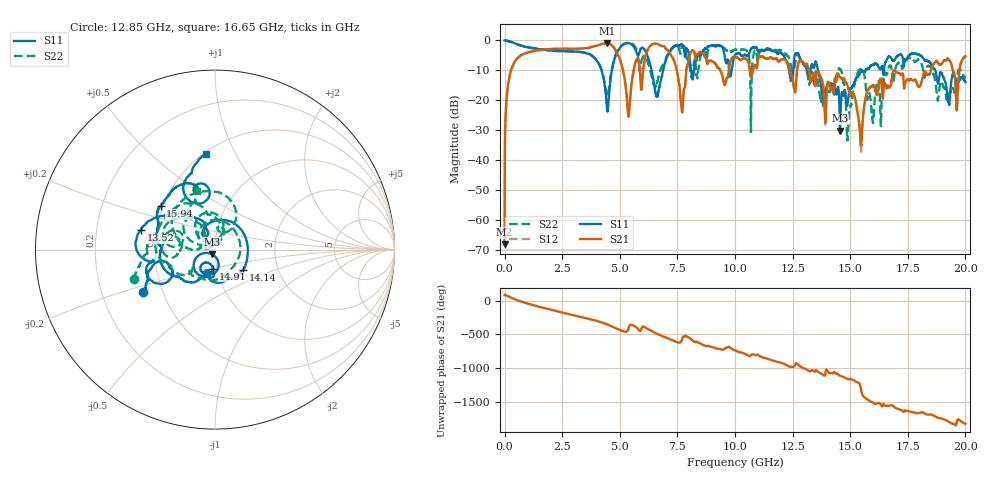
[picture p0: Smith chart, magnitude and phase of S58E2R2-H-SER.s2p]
!{S58E2R2}
!Johanson Technology Inc.
!www.johansontechnology.com
!Test Board Conditions:
!Substrate Type  RO4350B
!Substrate Thickness  60 mil
!Substrate Dk  3.66
!TL Type: GCPW
!TL Trace Width  115 mil
!TL Gap  52 mil
!Electrode orientation  Horizontal
!DUT TOPOLOGY	SERIES
!Mounting Pad LxW  55x428 mil
! Created Tue Apr 13 22:29:26 2021
# hz S ma R 50
! 2 Port Network Data from SP1.SP block
! freq  magS11  angS11  magS21  angS21  magS12  angS12  magS22  angS22
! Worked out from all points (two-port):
!   20001 points, 300 kHz to 20 GHz, reference 50 ohm
!   highest |S21| = -0.92 dB at 4.441 GHz (marker M1); lowest = -68.0 dB at 300 kHz (marker M2)
!   |S21| within 3 dB of the highest: 1.034 GHz to 4.866 GHz (3.832 GHz wide, 130 % of centre); 6.16 GHz to 7.152 GHz (992.1 MHz wide, 14.9 % of centre)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
!   lowest |S11| = -30.1 dB at 14.56 GHz (marker M3), VSWR 1.06, Z = 48.1 - j2.42 ohm
!   |S11| at or under -10 dB: 6.38 GHz to 6.879 GHz (498.7 MHz wide, 7.52 % of centre); 13.61 GHz to 15.66 GHz (2.057 GHz wide, 14.1 % of centre); 18.69 GHz to end of sweep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
!   |S22| runs from -33.3 to 0.0 dB; largest |S21 - S12| = 0.0083
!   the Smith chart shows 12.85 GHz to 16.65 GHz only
!   S11 on the Smith chart (normalised r, x): 12.85 GHz: 0.39, -0.24; 13.52 GHz: 0.41, +0.11; 14.14 GHz: 1.33, -0.32; 14.91 GHz: 0.96, -0.20; 15.94 GHz: 0.48, +0.28; 16.65 GHz: 0.52, +0.77
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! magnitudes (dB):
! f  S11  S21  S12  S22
! 300 kHz  0.0  -68.0  -68.6  0.0
! 124.3 MHz  -0.1  -16.3  -16.3  -0.1
! 428.3 MHz  -0.9  -7.2  -7.2  -0.9
! 3.334 GHz  -3.9  -2.7  -2.7  -3.9
! 4.441 GHz  -22.4  -0.9  -0.9  -18.5
! 5.376 GHz  -0.9  -25.4  -25.5  -0.8
! 6.667 GHz  -17.4  -1.3  -1.3  -12.6
! 7.699 GHz  -1.4  -23.8  -23.7  -1.9
! 8.128 GHz  -12.3  -3.3  -3.3  -11.9
! 10 GHz  -4.9  -5.5  -5.5  -3.1
! 12.85 GHz  -6.6  -6.7  -6.7  -6.3
! 13.33 GHz  -7.9  -13.3  -13.1  -10.7
! 13.52 GHz  -7.4  -12.2  -12.1  -10.6
! 14.14 GHz  -14.3  -15.8  -16.0  -16.5
! 14.56 GHz  -30.1  -12.3  -12.2  -9.6
! 14.91 GHz  -19.4  -15.8  -15.8  -29.3
! 15.46 GHz  -10.4  -34.1  -35.7  -9.5
! 15.94 GHz  -8.2  -15.2  -15.4  -24.2
! 16.65 GHz  -5.4  -15.3  -15.3  -9.4
! 16.67 GHz  -5.4  -15.5  -15.5  -9.0
! 19.63 GHz  -14.0  -23.2  -23.2  -12.1
! 20 GHz  -13.9  -5.3  -5.3  -12.3
